(* Logix 5000 AddOnInstructionDefinition export V430_Copy_Input_Small_100; software revision 33.01 *)

TYPE INPUT_Small_100 :
STRUCT
   User_Tag_Echo : DINT;
   Command : V430_100_101_Command_Echo;
   Output_Cmd : V430_100_101_Ext_Output_Echo;
   Read_Cycle_Sequence_Counter : DINT;
   Decode_Data : V430_Small_64_Char_Str;
END_STRUCT
END_TYPE

TYPE OUTPUT_198 :
STRUCT
   UserTag : DINT;
   Commands : V430_198_Commands;
   Ext_Outputs : V430_198_Ext_Output;
END_STRUCT
END_TYPE

TYPE V430_100_101_Command_Echo :
STRUCT
   Trigger_Echo : BOOL;
   New_Master_Echo : BOOL;
   Reserved01 : BOOL;
   Reserved02 : BOOL;
   Reserved03 : BOOL;
   Reserved04 : BOOL;
   Reserved05 : BOOL;
   Reserved06 : BOOL;
   Disable_Scanning_Echo : BOOL;
   Reserved07 : BOOL;
   Reserved08 : BOOL;
   Reserved09 : BOOL;
   Reserved10 : BOOL;
   Reserved11 : BOOL;
   Reserved12 : BOOL;
   Reserved13 : BOOL;
   Clear_Read_Cycle_Report_and_Counts_Echo : BOOL;
   Unlatch_Outputs_Echo : BOOL;
   Reserved14 : BOOL;
   Reserved15 : BOOL;
   Reserved16 : BOOL;
   Reserved17 : BOOL;
   Reserved18 : BOOL;
   Reserved19 : BOOL;
   Reserved : SINT;
END_STRUCT
END_TYPE

TYPE V430_100_101_Ext_Output_Echo :
STRUCT
   Output1_Echo : BOOL;
   Output2_Echo : BOOL;
   Output3_Echo : BOOL;
   Reserved01 : BOOL;
   Reserved02 : BOOL;
   Reserved03 : BOOL;
   Reserved04 : BOOL;
   Reserved05 : BOOL;
   Reserved06 : INT;
END_STRUCT
END_TYPE

TYPE V430_198_Commands :
STRUCT
   Trigger : BOOL;
   New_Master : BOOL;
   Reserved01 : BOOL;
   Reserved02 : BOOL;
   Reserved03 : BOOL;
   Reserved04 : BOOL;
   Reserved05 : BOOL;
   Reserved06 : BOOL;
   Disable_Scanning : BOOL;
   Reserved07 : BOOL;
   Reserved08 : BOOL;
   Reserved09 : BOOL;
   Reserved10 : BOOL;
   Reserved11 : BOOL;
   Reserved12 : BOOL;
   Reserved13 : BOOL;
   Clear_Read_Cycle_Report_and_Counters : BOOL;
   Unlatch_Outputs : BOOL;
   Reserved14 : BOOL;
   Reserved15 : BOOL;
   Reserved16 : BOOL;
   Reserved17 : BOOL;
   Reserved18 : BOOL;
   Reserved19 : BOOL;
   Reserved : SINT;
END_STRUCT
END_TYPE

TYPE V430_198_Ext_Output :
STRUCT
   Output1 : BOOL;
   Output2 : BOOL;
   Output3 : BOOL;
   Reserved01 : BOOL;
   Reserved02 : BOOL;
   Reserved03 : BOOL;
   Reserved04 : BOOL;
   Reserved05 : BOOL;
   Reserved06 : INT;
END_STRUCT
END_TYPE

TYPE V430_Small_64_Char_Str :   // string type
STRUCT
   LEN : DINT;
   DATA : SINT[64];
END_STRUCT
END_TYPE

ADD_ON_INSTRUCTION V430_Copy_Input_Small_100   (* revision 1.0, vendor OMRON *)
// Copies Omron V430-F reader EtherNet/IP input and output assemblies to local tags.
// Requires use of Input Small (100) and Output (198) assemblies.
VAR_IN_OUT
   Assembly_Input : INPUT_Small_100; {required}   // User MicroHAWK Input Assembly
   Assembly_Output : OUTPUT_198; {required}   // User MicroHAWK Output Assembly
   Connection_Input : SINT[84]; {required}   // EIP Input Connection
   Connection_Output : SINT[12]; {required}   // EIP Output Connection
END_VAR

ROUTINE Logic   (* ladder *)
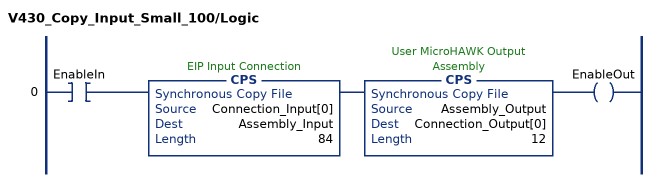
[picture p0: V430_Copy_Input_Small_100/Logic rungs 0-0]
   0: XIC(EnableIn)CPS(Connection_Input[0],Assembly_Input,84)CPS(Assembly_Output,Connection_Output[0],12)OTE(EnableOut);
END_ROUTINE
END_ADD_ON_INSTRUCTION
